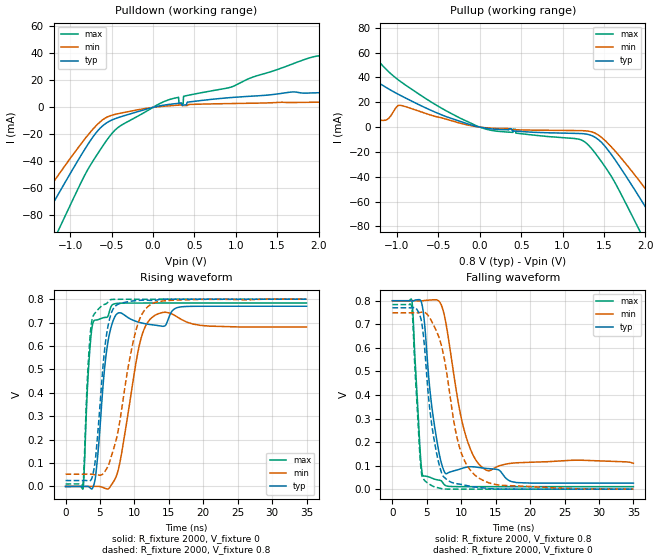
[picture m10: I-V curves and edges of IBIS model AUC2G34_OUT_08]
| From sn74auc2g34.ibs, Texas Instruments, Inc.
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[Model]   AUC2G34_OUT_08
Model_type  Output
Vref =   0
Rref =   2000
Cref =   15p
Vmeas =   0.4
| variable   typ   min   max
C_comp   5.70pF   2.73pF   7.64pF
| C_pullup   5.16pF   2.73pF   7.64pF
| C_pulldown   6.24pF   5.45pF   6.86pF
[Temperature Range]   40   100   -40
| Ambient temperature   25   85   -40
[Voltage range]   0.8   0.8   0.8
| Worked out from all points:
|   slope of the pulldown table from 0 to 0.12 V, typ, clamps not added: 77.1 ohm
|   slope of the pullup table from 0 to 0.12 V, typ, clamps not added: 92.7 ohm
|   rising waveform, R_fixture 2000, V_fixture 0: 20-80 % time 1.41ns typ, 2.22ns min, 824ps max; typ from 0 V to 0.77 V
|   falling waveform, R_fixture 2000, V_fixture 0.8: 20-80 % time 1.77ns typ, 2.44ns min, 874ps max; typ from 0.8 V to 0.026 V
|   rising waveform, R_fixture 2000, V_fixture 0.8: 20-80 % time 1.39ns typ, 2.71ns min, 771ps max; typ from 0.025 V to 0.8 V
|   falling waveform, R_fixture 2000, V_fixture 0: 20-80 % time 1.78ns typ, 2.85ns min, 867ps max; typ from 0.77 V to 0 V
[Pulldown]
| AUC2G34_OUT_08
|   Voltage   I(typ)   I(min)   I(max)
-3.6V     -332.4mA   -278mA     -406.9mA
-1.635V   -117.6mA   -94.31mA   -155.4mA
-1.375V   -89.36mA   -70.77mA   -121.6mA
-1.155V   -65.66mA   -51.28mA   -92.93mA
-630mV    -14.96mA   -10.34mA   -30.86mA
-430mV    -7.788mA   -4.787mA   -15.33mA
-90mV     -1.494mA   -794.3uA   -3.292mA
210mV     2.329mA    1.254mA    6.027mA
365mV     1.692mA    1.285mA    2.781mA
1.98V     10.84mA    3.867mA    38.03mA
2.365V    11.74mA    4.199mA    33.49mA
7.2V      23.85mA    8.894mA    59.34mA
[Pullup]
| AUC2G34_OUT_08
|   Voltage   I(typ)   I(min)   I(max)
-3.6V     79.22mA    9.067mA    184.4mA
-3.085V   77.82mA    9.388mA    162mA
-1.585V   27.55mA    10.91mA    82.21mA
-1.305V   38.3mA     6.636mA    59.53mA
-1.13V    31.96mA    5.757mA    46.56mA
-975mV    26.16mA    17.62mA    37.64mA
-235mV    4.613mA    3.12mA     7.149mA
1.36V     -7.061mA   -3.968mA   -18.09mA
1.87V     -50.43mA   -38.4mA    -75.48mA
2.115V    -76.59mA   -59.64mA   -107.9mA
2.4V      -107.6mA   -85.19mA   -145.4mA
7.2V      -634.6mA   -538mA     -765.9mA
[Ramp]
| AUC2G34_OUT_08
| variable   typ   min   max
dV/dt_r   0.47/1.42E-09   0.45/2.51E-09   0.48/8.28E-10
dV/dt_f   0.47/1.78E-09   0.44/2.66E-09   0.48/8.80E-10
R_load = 2000
[Rising Waveform]
| AUC2G34_OUT_08
R_fixture =   2000
C_fixture =   0
L_fixture =   0
V_fixture =   0
V_fixture_min = 0
V_fixture_max = 0
|   Time   V(typ)   V(min)   V(max)
0s        8.052nV    45.46nV    527.4pV
2.555ns   176uV      -48.11uV   -7.112mV
3.375ns   -1.45mV    207.8uV    523mV
4.155ns   11.36mV    553.5uV    709.1mV
5.8ns     541.6mV    -8.578mV   722.4mV
6.82ns    701.1mV    14.07mV    776.9mV
7.925ns   741.8mV    107.4mV    782.9mV
10.81ns   700.3mV    615mV      783.6mV
12.65ns   690.5mV    724.3mV    783.7mV
34.99ns   770mV      681mV      783.8mV
[Falling Waveform]
| AUC2G34_OUT_08
R_fixture =   2000
C_fixture =   0
L_fixture =   0
V_fixture =   0.8
V_fixture_min = 0.8
V_fixture_max = 0.8
|   Time   V(typ)   V(min)   V(max)
0s        800mV      800mV      800mV
2.84ns    798.7mV    800mV      796.5mV
4.045ns   802.9mV    798.9mV    151.8mV
4.425ns   762.1mV    799.9mV    56.71mV
5.87ns    317mV      803.8mV    45.17mV
7.715ns   66.37mV    712.6mV    15.27mV
10.32ns   90.17mV    261.5mV    10.7mV
13.19ns   89.52mV    89.01mV    10.65mV
18.08ns   27.93mV    112.1mV    10.63mV
34.99ns   25.52mV    109.9mV    10.61mV
[Rising Waveform]
| AUC2G34_OUT_08
R_fixture =   2000
C_fixture =   0
L_fixture =   0
V_fixture =   0.8
V_fixture_min = 0.8
V_fixture_max = 0.8
|   Time   V(typ)   V(min)   V(max)
0s        25.46mV    52.25mV    10.6mV
2.525ns   25.59mV    52.25mV    11.28mV
3.18ns    24.71mV    52.43mV    466.2mV
3.66ns    26.92mV    52.23mV    674.3mV
4.325ns   113.5mV    50.31mV    742.3mV
5.25ns    446.2mV    49.81mV    771.2mV
6.915ns   758.6mV    154.6mV    799.2mV
10.04ns   793.4mV    645.2mV    799.8mV
11.97ns   795.4mV    769.1mV    799.9mV
34.99ns   800mV      800.2mV    800mV
[Falling Waveform]
| AUC2G34_OUT_08
R_fixture =   2000
C_fixture =   0
L_fixture =   0
V_fixture =   0
V_fixture_min = 0
V_fixture_max = 0
|   Time   V(typ)   V(min)   V(max)
0s        770mV      748.6mV    783.8mV
2.775ns   769.5mV    748.5mV    775.6mV
4.09ns    728mV      750.5mV    104mV
4.52ns    645.7mV    751.6mV    42.6mV
4.965ns   488.7mV    744.7mV    29.31mV
5.835ns   249.1mV    704.6mV    13.07mV
7.23ns    61.96mV    595.8mV    1.601mV
9.585ns   22.08mV    194.1mV    89.44uV
12.11ns   8.441mV    56.04mV    50.61uV
34.99ns   38.75uV    32.14uV    11.58uV
